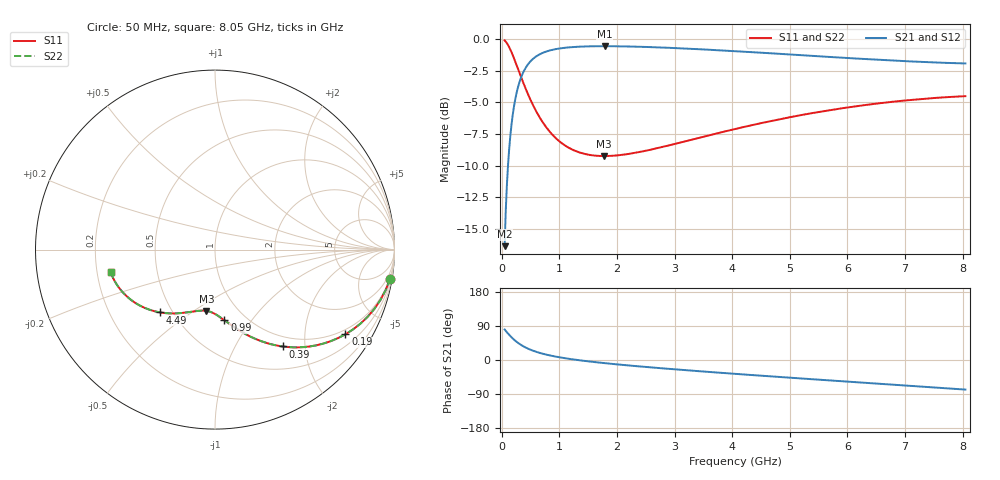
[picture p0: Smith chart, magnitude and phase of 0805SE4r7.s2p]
! AVX Thin Film Operation		Date: August 2001
! Description: Accu-P® Series, Thin Film, SMD, RF Capacitor
! Part Number: 08051J4R7ABT
! 50 MHz  -  8.05 GHz
! Serial Measurements
# mhz S db R 50
!	S11		S21		S12		S22
!	dB	Phase	dB	Phase	dB	Phase	dB	Phase
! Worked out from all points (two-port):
!   401 points, 50 MHz to 8.05 GHz, reference 50 ohm
!   highest |S21| = -0.55 dB at 1.79 GHz (marker M1); lowest = -16.4 dB at 50 MHz (marker M2)
!   |S21| within 3 dB of the highest: 297.8 MHz to end of sweep
!   lowest |S11| = -9.2 dB at 1.77 GHz (marker M3), VSWR 2.05, Z = 36.3 - j28.1 ohm
!   |S11| at or under -10 dB: nowhere
!   |S22| runs from -9.2 to -0.1 dB; largest |S21 - S12| = 0
!   S11 on the Smith chart (normalised r, x): 50 MHz: 1, -12; 190 MHz: 0.84, -3.17; 390 MHz: 0.83, -1.59; 990 MHz: 0.80, -0.75; 4.49 GHz: 0.43, -0.38; 8.05 GHz: 0.26, -0.10
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50  -0.10 -9.5  -16.38 80.5  -16.38 80.5  -0.10 -9.5
90  -0.32 -16.9  -11.51 73.1  -11.51 73.1  -0.32 -16.9
110  -0.47 -20.4  -9.92 69.6  -9.92 69.6  -0.47 -20.4
130  -0.64 -23.7  -8.66 66.2  -8.66 66.2  -0.64 -23.8
190  -1.25 -33.0  -6.03 57.0  -6.03 57.0  -1.25 -33.0
270  -2.19 -43.4  -4.02 46.6  -4.02 46.6  -2.19 -43.4
330  -2.92 -49.7  -3.10 40.3  -3.10 40.3  -2.92 -49.7
390  -3.63 -55.1  -2.47 34.9  -2.47 34.9  -3.63 -55.1
510  -4.91 -63.5  -1.70 26.5  -1.70 26.5  -4.91 -63.5
630  -5.97 -69.9  -1.27 20.1  -1.27 20.1  -5.97 -69.9
790  -7.07 -76.3  -0.95 13.6  -0.95 13.6  -7.07 -76.3
990  -8.04 -82.5  -0.74 7.5  -0.74 7.5  -8.04 -82.5
1390  -9.02 -91.4  -0.58 -1.5  -0.58 -1.5  -9.02 -91.4
1770  -9.25 -98.0  -0.55 -8.1  -0.55 -8.1  -9.25 -98.0
1790  -9.25 -98.3  -0.55 -8.4  -0.55 -8.4  -9.25 -98.3
2730  -8.60 -111.2  -0.65 -21.3  -0.65 -21.3  -8.60 -111.2
3370  -7.87 -118.8  -0.78 -28.9  -0.78 -28.9  -7.87 -118.8
4050  -7.11 -126.4  -0.95 -36.5  -0.95 -36.5  -7.11 -126.4
4490  -6.66 -131.2  -1.07 -41.3  -1.07 -41.3  -6.66 -131.2
5390  -5.85 -140.6  -1.32 -50.7  -1.32 -50.7  -5.85 -140.6
6730  -4.98 -154.3  -1.68 -64.4  -1.68 -64.4  -4.98 -154.3
8050  -4.51 -167.9  -1.92 -78.1  -1.92 -78.1  -4.51 -167.9
